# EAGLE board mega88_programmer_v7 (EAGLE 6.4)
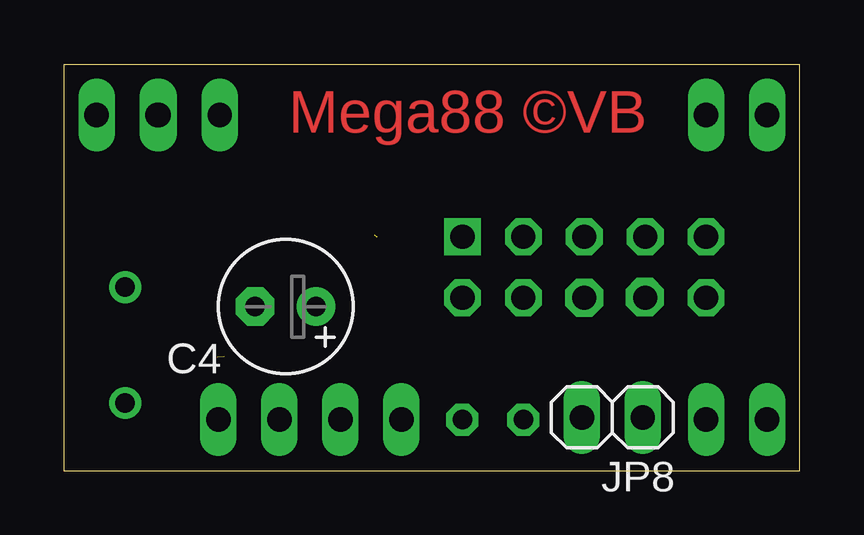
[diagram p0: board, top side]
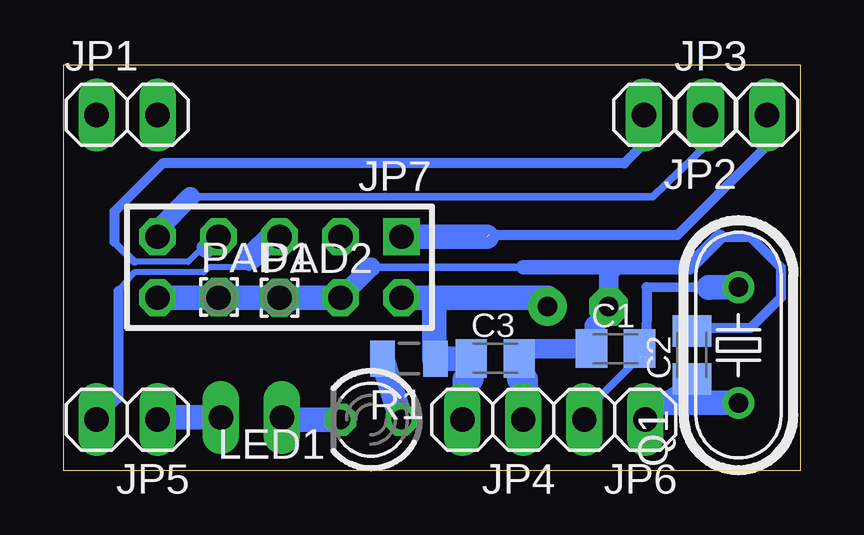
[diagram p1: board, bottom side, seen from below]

Size 30.67 x 16.92 mm. Coordinates in mm from the lower left corner, seen from the top.
Outline: 0,0 30.67,0 30.67,16.92 0,16.92 0,0
Copper layers (1*16): Top 0.035mm / dielectric 1.5mm / Bottom 0.035mm
Design rules "default": minimum track width 10mil, minimum drill 24mil, track to track 8mil, track to pad 8mil, pad to pad 8mil, via to via 8mil, smd to smd 8mil, copper to edge 40mil, drill to drill 8mil, minimum pad ring 10mil, minimum via ring 8mil, stop-mask expansion 4mil, vias tented up to drill 0mil, thermal gap 10mil

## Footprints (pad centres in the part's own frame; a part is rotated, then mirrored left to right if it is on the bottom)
C0805K = smd 1.3 x 1.6: 1 -1,0; 2 1,0
E2,5-6 = drill 0.813 pad 1.6: + -1.27,0 | drill 0.813 pad 1.6 octagon: - 1.27,0
1X02 = drill 1.016 long: 1 -1.27,0; 2 1.27,0
AVR-ISP-10 = drill 1.016 square: 1 -5.08,-1.27 | drill 1.016 octagon: 2 -5.08,1.27; 3 -2.54,-1.27; 4 -2.54,1.27; 5 0,-1.27; 6 0,1.27; 7 2.54,-1.27; 8 2.54,1.27; 9 5.08,-1.27; 10 5.08,1.27
LED3MM = drill 0.813 octagon: A -1.27,0; K 1.27,0
1,6/0,9 = drill 0.914 pad 1.6 octagon: 1 0,0
HC49U-V = drill 0.813: 1 -2.413,0; 2 2.413,0
R0805 = smd 1.016 x 1.5: 1 -1.109,0; 2 1.109,0

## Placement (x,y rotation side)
C1  [C0805K]  7.69,5.09 0 bottom
C2  [C0805K]  4.51,4.82 90 bottom
C3  [C0805K]  12.7,4.68 0 bottom
C4  [E2,5-6]  9.25,6.84 180 top
JP1  [1X02]  28.04,14.83 0 bottom
JP2  [1X02]  5.23,14.83 180 bottom
JP3  [1X02]  2.64,14.83 0 bottom
JP4  [1X02]  12.8,2.13 180 bottom
JP5  [1X02]  28.04,2.13 180 bottom
JP6  [1X02]  7.72,2.13 180 bottom
JP7  AVR-ISP-10  [AVR-ISP-10]  21.69,8.48 180 bottom
JP8  [1X02]  22.86,2.22 180 top
LED1  [LED3MM]  17.88,2.13 180 bottom
PAD1  WIREPAD1,6/0,9  [1,6/0,9]  24.21,7.24 0 bottom
PAD2  WIREPAD1,6/0,9  [1,6/0,9]  21.69,7.21 0 bottom
Q1  [HC49U-V]  2.57,5.24 90 bottom
R1  [R0805]  16.29,4.67 180 bottom

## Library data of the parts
C1-C4 R1 = rcl
JP1-JP6 JP8 = pinhead
JP7 = avr-6
LED1 = led
PAD1 PAD2 = wirepad
Q1 = crystal

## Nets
N$1: C3.1 C4.+ JP4.2 JP7.2 R1.1
N$2: C1.1 C2.2 C3.2 C4.- JP4.1 JP7.4 PAD2.1
N$3: JP5.2 JP7.5
N$4: JP2.2 JP7.7
N$5: JP3.1 JP7.9
N$6: JP3.2 JP7.1
N$7: C1.2 JP6.2 Q1.2
N$8: C2.1 JP6.1 Q1.1
N$9: JP5.1 JP8.1
N$10: LED1.A R1.2
N$11: JP7.6 JP7.8 JP7.10 PAD1.1
N$12: JP8.2 LED1.K

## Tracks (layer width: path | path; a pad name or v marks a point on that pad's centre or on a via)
N$1
  Bottom 1.016: JP7.2 15.24,7.21 | 15.24,7.21 10.52,7.21 C4.+ | 15.24,7.21 15.24,4.67 R1.1 13.7,4.67 C3.1 13.7,3.81 13.97,3.81 13.97,2.13 JP4.2
N$2
  Bottom 0.305: 17.88,8.48 11.53,8.48
  Bottom 0.406: 3.34,9.75 2.07,9.75 0.8,8.48 0.8,7.21 2.07,5.94 5.03,5.94 C2.2
  Bottom 0.61: 3.34,9.75 4.61,8.48 7.62,8.48 | 11.53,8.48 7.62,8.48 | 7.98,8.12 7.62,8.48
  Bottom 0.813: JP7.4 17.88,8.48 | 7.98,8.12 C4.- 7.98,6.63 8.57,6.03 8.57,5.2 C1.1 11.29,5.09 C3.2
  Bottom 1.016: JP4.1 11.43,2.13 11.43,3.81 11.7,3.81 C3.2 | PAD2.1 JP7.4
N$3
  Bottom 0.254: 22.96,8.48 24.64,8.48 24.86,8.26 27.74,8.26 28.4,7.5
  Bottom 0.305: 22.96,8.48 22.96,8.79 22.86,8.89
  Bottom 0.406: 28.4,7.5 28.4,3.04 JP5.2
  Bottom 1.016: JP7.5 22,9.75 22.86,8.89
N$4
  Bottom 0.254: 24.74,9.26 25,9.2 25.5,8.7 27.7,8.7
  Bottom 0.305: 27.7,8.7 27.75,8.7 28.57,9.53
  Bottom 0.406: JP2.2 6.45,13.68 7.32,12.81 26.56,12.81 28.57,10.79 28.57,9.53
  Bottom 0.813: JP7.7 24.25,9.75 24.74,9.26
N$5
  Bottom 0.254: JP7.9 26.77,9.7
  Bottom 0.305: JP3.1 3.91,13.56 6.14,11.41 25.4,11.41 25.4,11.43
  Bottom 0.813: JP7.9 26.77,10.04 25.4,11.41
N$6  (1 unrouted)
  Bottom 0.406: 12.95,9.83 5.1,9.83 1.37,13.56 JP3.2
  Bottom 1.016: JP7.1 13.05,9.75
N$7  (1 unrouted)
  Bottom 0.305: C1.2 6.69,4.74 8.89,2.54 8.89,2.23 JP6.2
  Bottom 0.406: 3.81,7.62 6.39,7.65 6.41,4.74
  Bottom 1.016: Q1.2 3.81,7.65 3.81,7.62
N$8
  Bottom 0.406: JP6.1 6.45,2.51 C2.1
  Bottom 1.016: Q1.1 6.07,2.82 6.35,2.54 6.35,2.23 JP6.1
N$9
  Bottom 1.016: JP8.1 26.77,2.22 JP5.1
N$10
  Bottom 1.016: LED1.A R1.2
N$11
  Bottom 1.016: JP7.10 JP7.8 | JP7.8 24.21,7.21 PAD1.1 | JP7.8 JP7.6
N$12
  Bottom 1.016: LED1.K 21.59,2.13 JP8.2

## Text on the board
Top: Mega88 ©VB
